|   TEXAS INSTRUMENTS INCORPORATED
|   Standard Linear and Logic
|   IBIS Model of SN74LVT16245B
|   3.3-V ABT 16-BIT BUS TRANSCEIVERS WITH 3-STATE OUTPUTS
|   TSSOP 48-pin (DGG) package
|   TVSOP 48-pin (DGV) package
|   SSOP 48-pin (DL) package
|   VFBGA 48-pin (GQL) package
[IBIS Ver]   3.2
[Comment Char]  |_char
[File Name]   sn74lvt16245b.ibs
[File Rev]   2.3 | e_die
[Date]   November 24, 2004
[Source]   File originated at Texas Instruments, Inc.
[Notes]   The following is a sample IBIS file for the SN74LVT16245B.
   - FILE REV HISTORY
   - 2.3 Re-Release IBIS file on 12/21/04
   - All test data contained in this file are derived from
   - All test data contained in this file are derived from
   actual measurement.
   - We have data across voltage and temperature, but not across
   process.
   - Since this is a BiCMOS process, we have irregular trend for the
   curves at high and low temperatures. This data was taken with
   high temperature for strong case and low for weak case.
   - Non-monotonic data in pullup as the device is
   overvoltage tolerant.
   - File created by Nobuhisa Ohtsubo, TIJ SLL Product Engineering.
|*   Property of Texas Instruments Incorporated.  Unauthorized   *
|*   reproduction and/or distribution is strictly prohibited.   *
|*   This product is protected under copyright law.   *
|*   Created 1998, (C) Copyright 1998, Texas Instruments Inc.,   *
|*   All Rights Reserved   *
|*   UNLESS THERE IS A SIGNED, WRITTEN AGREEMENT TO THE   *
|*   CONTRARY, TEXAS INSTRUMENTS ("TI") IS PROVIDING THE SPICE   *
|*   MODELS "AS IS" AND WITHOUT ANY WARRANTY, EXPRESSED OR   *
|*   IMPLIED.  TI assumes no liability for:   *
|*   1) the accuracy of the IBIS models provided to your   *
|*   company;   *
|*   2) the proper functioning of these IBIS models in your   *
|*   design or for any resulting applications; or   *
|*   3) infringement of patents, copyrights or intellectual   *
|*   property rights resulting from your use of these   *
|*   IBIS models.   *
|*   TI provides IBIS Models as a service to our customers.   *
|*   You and your company shall not distribute, sell or give   *
|*   these models to anyone else without prior written   *
|*   permission from TI.   *
|*   TI reserves the right to make changes to our products or   *
|*   to discontinue any semiconductor product or service   *
|*   without notice, and advises our customers to obtain the   *
|*   latest version of relevant information to verify, before   *
|*   placing orders, that the information being relied on is   *
|*   current.   *
|*   Please be aware that your receipt and use of the IBIS   *
|*   information provided shall serve as acceptance of these   *
|*   terms and conditions.  If you do not accept these terms,   *
|*   you should return or destroy the IBIS models and any   *
|*   other accompanying information immediately.   *
|   TSSOP 48-pin (DGG) package
[Component]   LVT16245B_DGG
[manufacturer]   Texas Instruments, Inc.
[Package]
|   typ   min   max
R_pkg   0.04   0.035   0.051
L_pkg   3.019nH   2.486nH   4.099nH
C_pkg   0.507pF   0.334pF   0.809pF
[Pin] signal_name   model_name   R_pin   L_pin   C_pin
1   1DIR   LVT16245B_CTRL   0.041   4.017nH   0.759pF
2   1B1   LVT16245B_IO   0.042   3.737nH   0.792pF
3   1B2   LVT16245B_IO   0.042   3.480nH   0.661pF
4   GND   GND   0.038   3.131nH   0.575pF
5   1B3   LVT16245B_IO   0.047   3.122nH   0.566pF
6   1B4   LVT16245B_IO   0.043   2.948nH   0.504pF
7   VCC   POWER   0.045   2.845nH   0.397pF
8   1B5   LVT16245B_IO   0.049   2.835nH   0.394pF
9   1B6   LVT16245B_IO   0.048   2.715nH   0.378pF
10   GND   GND   0.050   2.664nH   0.363pF
11   1B7   LVT16245B_IO   0.050   2.585nH   0.348pF
12   1B8   LVT16245B_IO   0.049   2.550nH   0.337pF
13   2B1   LVT16245B_IO   0.049   2.541nH   0.336pF
14   2B2   LVT16245B_IO   0.050   2.574nH   0.348pF
15   GND   GND   0.049   2.618nH   0.359pF
16   2B3   LVT16245B_IO   0.046   2.671nH   0.375pF
17   2B4   LVT16245B_IO   0.045   2.754nH   0.389pF
18   VCC   POWER   0.044   2.823nH   0.450pF
19   2B5   LVT16245B_IO   0.042   2.968nH   0.503pF
20   2B6   LVT16245B_IO   0.051   3.108nH   0.535pF
21   GND   GND   0.042   3.175nH   0.587pF
22   2B7   LVT16245B_IO   0.041   3.449nH   0.678pF
23   2B8   LVT16245B_IO   0.044   3.766nH   0.804pF
24   2DIR   LVT16245B_CTRL   0.043   4.065nH   0.761pF
25   2NOE   LVT16245B_CTRL   0.041   3.994nH   0.757pF
26   2A8   LVT16245B_IO   0.039   3.649nH   0.789pF
27   2A7   LVT16245B_IO   0.038   3.362nH   0.660pF
28   GND   GND   0.038   3.082nH   0.574pF
29   2A6   LVT16245B_IO   0.044   2.990nH   0.522pF
30   2A5   LVT16245B_IO   0.041   2.917nH   0.495pF
31   VCC   POWER   0.043   2.820nH   0.448pF
32   2A4   LVT16245B_IO   0.043   2.699nH   0.385pF
33   2A3   LVT16245B_IO   0.045   2.628nH   0.372pF
34   GND   GND   0.046   2.556nH   0.356pF
35   2A2   LVT16245B_IO   0.046   2.495nH   0.344pF
36   2A1   LVT16245B_IO   0.047   2.487nH   0.334pF
37   1A8   LVT16245B_IO   0.047   2.490nH   0.335pF
38   1A7   LVT16245B_IO   0.046   2.486nH   0.343pF
39   GND   GND   0.045   2.566nH   0.356pF
40   1A6   LVT16245B_IO   0.044   2.639nH   0.374pF
41   1A5   LVT16245B_IO   0.043   2.701nH   0.386pF
42   VCC   POWER   0.043   2.817nH   0.450pF
43   1A4   LVT16245B_IO   0.041   2.935nH   0.501pF
44   1A3   LVT16245B_IO   0.047   3.035nH   0.529pF
45   GND   GND   0.043   3.171nH   0.589pF
46   1A2   LVT16245B_IO   0.040   3.415nH   0.682pF
47   1A1   LVT16245B_IO   0.043   3.741nH   0.809pF
48   1NOE   LVT16245B_CTRL   0.044   4.099nH   0.764pF
|   TVSOP 48-pin (DGV) package
[Component]   LVT16245B_DGV
[manufacturer]   Texas Instruments, Inc.
[Package]
|   typ   min   max
R_pkg   0.063   0.043   0.09
L_pkg   3.077nH   2.377nH   4.305nH
C_pkg   0.387pF   0.281pF   0.565pF
[Pin] signal_name   model_name   R_pin   L_pin   C_pin
1   1DIR   LVT16245B_CTRL   0.082   4.277nH   0.562pF
2   1B1   LVT16245B_IO   0.090   4.020nH   0.554pF
3   1B2   LVT16245B_IO   0.087   3.719nH   0.478pF
4   GND   GND   0.087   3.456nH   0.417pF
5   1B3   LVT16245B_IO   0.076   3.207nH   0.411pF
6   1B4   LVT16245B_IO   0.044   2.929nH   0.390pF
7   VCC   POWER   0.046   2.803nH   0.335pF
8   1B5   LVT16245B_IO   0.047   2.683nH   0.321pF
9   1B6   LVT16245B_IO   0.048   2.579nH   0.311pF
10   GND   GND   0.049   2.505nH   0.302pF
11   1B7   LVT16245B_IO   0.048   2.400nH   0.289pF
12   1B8   LVT16245B_IO   0.051   2.400nH   0.283pF
13   2B1   LVT16245B_IO   0.051   2.400nH   0.283pF
14   2B2   LVT16245B_IO   0.050   2.433nH   0.291pF
15   GND   GND   0.048   2.460nH   0.298pF
16   2B3   LVT16245B_IO   0.048   2.585nH   0.312pF
17   2B4   LVT16245B_IO   0.046   2.652nH   0.319pF
18   VCC   POWER   0.045   2.787nH   0.336pF
19   2B5   LVT16245B_IO   0.046   2.962nH   0.394pF
20   2B6   LVT16245B_IO   0.074   3.208nH   0.409pF
21   GND   GND   0.087   3.488nH   0.417pF
22   2B7   LVT16245B_IO   0.087   3.741nH   0.478pF
23   2B8   LVT16245B_IO   0.089   3.990nH   0.546pF
24   2DIR   LVT16245B_CTRL   0.084   4.305nH   0.557pF
25   2NOE   LVT16245B_CTRL   0.082   4.286nH   0.565pF
26   2A8   LVT16245B_IO   0.086   3.933nH   0.554pF
27   2A7   LVT16245B_IO   0.086   3.699nH   0.475pF
28   GND   GND   0.089   3.522nH   0.420pF
29   2A6   LVT16245B_IO   0.079   3.234nH   0.413pF
30   2A5   LVT16245B_IO   0.043   2.880nH   0.385pF
31   VCC   POWER   0.045   2.779nH   0.332pF
32   2A4   LVT16245B_IO   0.045   2.636nH   0.317pF
33   2A3   LVT16245B_IO   0.047   2.553nH   0.309pF
34   GND   GND   0.048   2.468nH   0.298pF
35   2A2   LVT16245B_IO   0.050   2.424nH   0.290pF
36   2A1   LVT16245B_IO   0.050   2.377nH   0.281pF
37   1A8   LVT16245B_IO   0.050   2.387nH   0.281pF
38   1A7   LVT16245B_IO   0.050   2.431nH   0.290pF
39   GND   GND   0.048   2.475nH   0.299pF
40   1A6   LVT16245B_IO   0.048   2.557nH   0.309pF
41   1A5   LVT16245B_IO   0.047   2.671nH   0.319pF
42   VCC   POWER   0.046   2.804nH   0.334pF
43   1A4   LVT16245B_IO   0.044   2.935nH   0.390pF
44   1A3   LVT16245B_IO   0.074   3.203nH   0.412pF
45   GND   GND   0.085   3.444nH   0.416pF
46   1A2   LVT16245B_IO   0.085   3.723nH   0.477pF
47   1A1   LVT16245B_IO   0.090   4.012nH   0.547pF
48   1NOE   LVT16245B_CTRL   0.083   4.288nH   0.558pF
|   SSOP 48-pin (DL) package
[Component]   LVT16245B_DL
[manufacturer]   Texas Instruments, Inc.
[Package]
|   typ   min   max
R_pkg   0.048   0.038   0.053
L_pkg   6.046nH   5.084nH   7.968nH
C_pkg   0.813pF   0.569pF   1.157pF
[Pin] signal_name   model_name   R_pin   L_pin   C_pin
 1   1DIR   LVT16245B_CTRL   0.046   7.968nH   1.017pF
 2   1B1   LVT16245B_IO   0.044   7.299nH   1.157pF
 3   1B2   LVT16245B_IO   0.043   6.765nH   1.058pF
 4   GND   GND   0.041   6.269nH   0.933pF
 5   1B3   LVT16245B_IO   0.038   5.856nH   0.829pF
 6   1B4   LVT16245B_IO   0.046   5.802nH   0.790pF
 7   VCC   POWER   0.050   5.656nH   0.738pF
 8   1B5   LVT16245B_IO   0.053   5.500nH   0.643pF
 9   1B6   LVT16245B_IO   0.052   5.304nH   0.606pF
10   GND   GND   0.053   5.189nH   0.583pF
11   1B7   LVT16245B_IO   0.051   5.084nH   0.569pF
12   1B8   LVT16245B_IO   0.053   5.862nH   0.833pF
13   2B1   LVT16245B_IO   0.053   5.862nH   0.833pF
14   2B2   LVT16245B_IO   0.051   5.084nH   0.569pF
15   GND   GND   0.053   5.189nH   0.583pF
16   2B3   LVT16245B_IO   0.052   5.304nH   0.606pF
17   2B4   LVT16245B_IO   0.053   5.500nH   0.643pF
18   VCC   POWER   0.050   5.656nH   0.738pF
19   2B5   LVT16245B_IO   0.046   5.802nH   0.790pF
20   2B6   LVT16245B_IO   0.038   5.856nH   0.829pF
21   GND   GND   0.041   6.269nH   0.933pF
22   2B7   LVT16245B_IO   0.043   6.765nH   1.058pF
23   2B8   LVT16245B_IO   0.044   7.299nH   1.157pF
24   2DIR   LVT16245B_CTRL   0.046   7.968nH   1.017pF
25   2NOE   LVT16245B_CTRL   0.046   7.968nH   1.017pF
26   2A8   LVT16245B_IO   0.044   7.299nH   1.157pF
27   2A7   LVT16245B_IO   0.043   6.765nH   1.058pF
28   GND   GND   0.041   6.269nH   0.933pF
29   2A6   LVT16245B_IO   0.038   5.856nH   0.829pF
30   2A5   LVT16245B_IO   0.046   5.802nH   0.790pF
31   VCC   POWER   0.050   5.656nH   0.738pF
32   2A4   LVT16245B_IO   0.053   5.500nH   0.643pF
33   2A3   LVT16245B_IO   0.052   5.304nH   0.606pF
34   GND   GND   0.053   5.189nH   0.583pF
35   2A2   LVT16245B_IO   0.051   5.084nH   0.569pF
36   2A1   LVT16245B_IO   0.053   5.862nH   0.833pF
37   1A8   LVT16245B_IO   0.053   5.862nH   0.833pF
38   1A7   LVT16245B_IO   0.051   5.084nH   0.569pF
39   GND   GND   0.053   5.189nH   0.583pF
40   1A6   LVT16245B_IO   0.052   5.304nH   0.606pF
41   1A5   LVT16245B_IO   0.053   5.500nH   0.643pF
42   VCC   POWER   0.005   5.656nH   0.738pF
43   1A4   LVT16245B_IO   0.046   5.802nH   0.790pF
44   1A3   LVT16245B_IO   0.038   5.856nH   0.829pF
45   GND   GND   0.041   6.269nH   0.933pF
46   1A2   LVT16245B_IO   0.043   6.765nH   1.058pF
47   1A1   LVT16245B_IO   0.044   7.299nH   1.157pF
48   1NOE   LVT16245B_CTRL   0.046   7.967nH   1.017pF
|   VFBGA 48-pin (GQL) package
[Component]   LVT16245B_GQL
[Manufacturer]   Texas Instruments, Inc.
[Package]
|   typ   min   max
R_pkg   7.900e-02   4.500e-02   9.400e-02
L_pkg   2.264e-09   1.398e-09   2.722e-09
C_pkg   3.060e-13   1.170e-13   4.040e-13
[Pin] signal_name  model_name   R_pin   L_pin   C_pin
A1   1DIR   LVT16245B_CTRL   5.100e-02   1.531e-09   2.100e-13
B2   1B1   LVT16245B_IO   7.300e-02   2.572e-09   3.120e-13
B1   1B2   LVT16245B_IO   7.100e-02   1.835e-09   2.320e-13
B3   GND   GND   9.400e-02   2.717e-09   3.830e-13
C2   1B3   LVT16245B_IO   8.900e-02   2.534e-09   3.500e-13
C1   1B4   LVT16245B_IO   7.100e-02   1.831e-09   2.310e-13
C3   VCC   POWER   9.400e-02   2.722e-09   3.920e-13
D2   1B5   LVT16245B_IO   9.000e-02   2.551e-09   3.520e-13
D1   1B6   LVT16245B_IO   7.200e-02   1.846e-09   2.440e-13
D3   GND   GND   9.400e-02   2.719e-09   4.030e-13
E2   1B7   LVT16245B_IO   8.900e-02   2.541e-09   3.510e-13
E1   1B8   LVT16245B_IO   7.200e-02   1.850e-09   2.270e-13
F1   2B1   LVT16245B_IO   7.200e-02   1.850e-09   2.270e-13
F2   2B2   LVT16245B_IO   8.900e-02   2.541e-09   3.510e-13
G3   GND   GND   9.400e-02   2.718e-09   4.040e-13
G1   2B3   LVT16245B_IO   7.200e-02   1.847e-09   2.440e-13
G2   2B4   LVT16245B_IO   9.000e-02   2.551e-09   3.520e-13
H3   VCC   POWER   9.400e-02   2.721e-09   3.920e-13
H1   2B5   LVT16245B_IO   7.000e-02   1.830e-09   2.310e-13
H2   2B6   LVT16245B_IO   8.800e-02   2.524e-09   3.500e-13
J3   GND   GND   9.300e-02   2.709e-09   3.820e-13
J1   2B7   LVT16245B_IO   7.100e-02   1.851e-09   2.330e-13
J2   2B8   LVT16245B_IO   5.600e-02   2.605e-09   3.900e-13
K1   2DIR   LVT16245B_CTRL   4.500e-02   1.398e-09   1.170e-13
K6   2NOE   LVT16245B_CTRL   4.500e-02   1.512e-09   1.930e-13
J5   2A8   LVT16245B_IO   5.500e-02   2.492e-09   3.130e-13
J6   2A7   LVT16245B_IO   7.000e-02   1.821e-09   2.300e-13
J4   GND   GND   9.300e-02   2.703e-09   3.820e-13
H5   2A6   LVT16245B_IO   8.900e-02   2.529e-09   3.500e-13
H6   2A5   LVT16245B_IO   7.100e-02   1.826e-09   2.300e-13
H4   VCC   POWER   9.400e-02   2.722e-09   3.910e-13
G5   2A4   LVT16245B_IO   9.000e-02   2.551e-09   3.520e-13
G6   2A3   LVT16245B_IO   7.200e-02   1.846e-09   2.440e-13
G4   GND   GND   9.400e-02   2.719e-09   4.040e-13
F5   2A2   LVT16245B_IO   8.800e-02   2.510e-09   3.490e-13
F6   2A1   LVT16245B_IO   7.200e-02   1.850e-09   2.270e-13
E6   1A8   LVT16245B_IO   7.100e-02   1.850e-09   2.270e-13
E5   1A7   LVT16245B_IO   8.900e-02   2.529e-09   3.500e-13
D4   GND   GND   9.400e-02   2.719e-09   4.030e-13
D6   1A6   LVT16245B_IO   7.200e-02   1.847e-09   2.430e-13
D5   1A5   LVT16245B_IO   8.900e-02   2.550e-09   3.520e-13
C4   VCC   POWER   9.400e-02   2.722e-09   3.910e-13
C6   1A4   LVT16245B_IO   7.100e-02   1.827e-09   2.300e-13
C5   1A3   LVT16245B_IO   8.900e-02   2.539e-09   3.500e-13
B4   GND   GND   9.300e-02   2.705e-09   3.820e-13
B6   1A2   LVT16245B_IO   7.100e-02   1.831e-09   2.270e-13
B5   1A1   LVT16245B_IO   7.300e-02   2.685e-09   3.800e-13
A6   1NOE   LVT16245B_CTRL   5.100e-02   1.417e-09   1.330e-13
[Model Selector]   LVT16245B_CTRL
LVT16245B_CTRL_28   2.8-V Vcc Input Model
LVT16245B_CTRL_33   3.3-V Vcc Input Model
[Model Selector]   LVT16245B_IO
LVT16245B_IO_28   2.8-V Vcc Input/Output Model
LVT16245B_IO_33   3.3-V Vcc Input/Output Model
| Models and submodels in the file (4): LVT16245B_IO_28 (I/O), LVT16245B_CTRL_28 (Input), LVT16245B_IO_33 (I/O), LVT16245B_CTRL_33 (Input)
